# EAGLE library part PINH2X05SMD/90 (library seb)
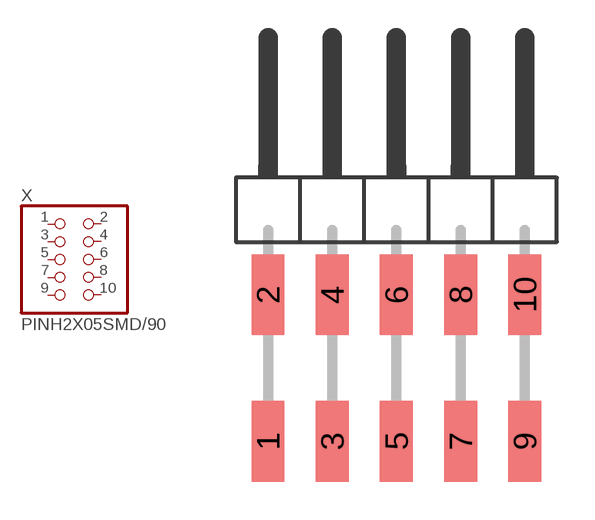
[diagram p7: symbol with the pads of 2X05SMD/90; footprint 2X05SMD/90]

Designator prefix X

## PINH2X05SMD/90  [2X05SMD/90]
1  1  pas
2  2  pas
3  3  pas
4  4  pas
5  5  pas
6  6  pas
7  7  pas
8  8  pas
9  9  pas
10  10  pas

## Footprint 2X05SMD/90 (pad centres in mm)
PIN HEADER - 2.54 90°
smd 1.3 x 3.2: 1 -1.27,-10.9; 2 -1.27,-5.1; 3 1.27,-10.9; 4 1.27,-5.1; 5 3.81,-10.9; 6 3.81,-5.1; 7 6.35,-10.9; 8 6.35,-5.1; 9 8.89,-10.9; 10 8.89,-5.1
